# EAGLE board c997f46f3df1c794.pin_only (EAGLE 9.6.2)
REV: C

Size 80.01 x 53.34 mm. Coordinates in mm from the lower left corner, seen from the top.
Outline: 2.41,53.34 77.34,53.34 arc-90 80.01,50.93 80.01,36.32 78.23,34.92 78.23,17.27 80.01,16.13 80.01,2.54 arc-90 77.47,0 2.53,0 arc-90 0,2.53 0,50.93 arc-90 2.41,53.34
Copper layers (1*16): Top 0.035mm / dielectric 1.5mm / Bottom 0.035mm
Design rules "adafruit *": minimum track width 8mil, minimum drill 15.5mil, track to track 8mil, track to pad 8mil, pad to pad 8mil, via to via 8mil, smd to smd 8mil, copper to edge 10mil, drill to drill 8mil, minimum pad ring 10mil, minimum via ring 8mil, stop-mask expansion 2mil, vias tented up to drill 20mil, thermal gap 10mil
Net classes: 0 default: width 0.178 mm; 1 power: width 0.254 mm; 2 lowpower: width 0.305 mm, drill 0.483 mm

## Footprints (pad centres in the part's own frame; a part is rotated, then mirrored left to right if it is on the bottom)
0805-NO = smd 1.24 x 1.5: 1 -0.95,0; 2 0.95,0
0603-NO = smd 1.075 x 1: 1 -0.85,0; 2 0.85,0
CHIPLED_0603_NOOUTLINE = smd 0.8 x 0.8: A 0,-0.75; C 0,0.75
JST_SH4 = smd 0.6 x 1.55: 1 -1.5,2.514; 2 -0.5,2.514; 3 0.5,2.514; 4 1.5,2.514 | smd 1.2 x 1.8: MT1 -2.8,-1.386; MT2 2.8,-1.386
SOD-323 = smd 1.35 x 0.8: A 1.27,0; C -1.27,0
SOD-123 = smd 1.4 x 1.4: A 1.85,0; C -1.85,0
EINK_290IN = smd 1.25 x 0.275 bottom: 1 2.51,5.208; 2 2.51,4.708; 3 2.51,4.208; 4 2.51,3.708; 5 2.51,3.208; 6 2.51,2.708; 7 2.51,2.208; 8 2.51,1.708; 9 2.51,1.208; 10 2.51,0.708; 11 2.51,0.208; 12 2.51,-0.292; 13 2.51,-0.792; 14 2.51,-1.292; 15 2.51,-1.792; 16 2.51,-2.292; 17 2.51,-2.792; 18 2.51,-3.292; 19 2.51,-3.792; 20 2.51,-4.292; 21 2.51,-4.792; 22 2.51,-5.292; 23 2.51,-5.792; 24 2.51,-6.292 | smd 3 x 2 bottom: SPRT1 0.05,7.058; SPRT2 0.05,-8.052
FIDUCIAL_1MM = smd 1 x 1: 1 0,0
SOT23-6 = smd 0.55 x 1.2: 1 -0.95,-1.3; 2 0,-1.3; 3 0.95,-1.3; 4 0.95,1.3; 5 0,1.3; 6 -0.95,1.3
LGA16_3X3MM = smd 0.5 x 0.25: 1 -1.35,1; 2 -1.35,0.5; 3 -1.35,0; 4 -1.35,-0.5; 5 -1.35,-1; 9 1.35,-1; 10 1.35,-0.5; 11 1.35,0; 12 1.35,0.5; 13 1.35,1 | smd 0.25 x 0.5: 6 -0.5,-1.35; 7 0,-1.35; 8 0.5,-1.35; 14 0.5,1.35; 15 0,1.35; 16 -0.5,1.35
1X02_ROUND = drill 1 pad 1.778: 1 -1.27,0; 2 1.27,0
INDUCTOR_4X4MM_NR401 = smd 1.2 x 3.7: P$1 -1.4,0; P$2 1.4,0
WS2812B_4020 = smd 0.5 x 1.25: 1 1.3,-0.75; 2 0.45,-0.75; 3 -0.45,-0.75; 4 -1.3,-0.75
SOT23-R = smd 0.635 x 1.016: 1 -0.95,-1; 2 0.95,-1; 3 0,1
SOT23-3 = smd 0.8 x 0.9: 1 -0.95,-1; 2 0.95,-1; 3 0,1.1
0805_10MGAP = smd 1.2 x 1.5: 1 -1.05,0; 2 1.05,0
JSTPH3 = smd 1 x 4.6: 1 -2,-2.7; 2 0,-2.7; 3 2,-2.7 | smd 1.6 x 3.4: NC1 -4.4,2.5; NC2 4.4,2.5
SOLDERJUMPER_2WAY_OPEN_NOPASTE = smd 1.168 x 1.6: 1 -1.397,0; 2 0,0; 3 1.397,0
BUZZER_SMT_7.5MM = smd 2 x 2: + 2.8,-2.8; - 2.8,2.8; MT2 -2.8,2.8 | smd 2 x 1 rotated 135: MT -3,-3
SPST_TACTILE_RA = smd 1.1 x 1.5: 1 -2.1,0.9; 2 2.1,0.9 | smd 1.75 x 1: MT1 -3.175,-0.9; MT2 3.075,-0.9 | hole 1: -1.15,-0.3; 1.15,-0.3
TACTILE_3X6MM = smd 2 x 1.5: P$1 -4,0; P$2 4,0
SPDT_SMT_SSSS811101 = smd 0.7 x 1.5: A -2.25,1.75; B 0.75,1.75; C 2.25,1.75 | smd 1 x 0.8: SUP1 -3.65,1.1; SUP2 -3.65,-1.1; SUP3 3.65,1.1; SUP4 3.65,-1.1 | hole 0.9: -1.5,0; 1.5,0
TESTPOINT_ROUND_1.5MM_NO = smd 1.5 x 1.5: P$1 0,0
SMT_NUT_3MM = drill 4.25 pad 4.572: P$1 0,0
ALS-PT19-315C = smd 0.8 x 0.8: C -0.75,0; E 0.75,0
SOT23-5 = smd 0.55 x 1.2: 1 -0.95,-1.3; 2 0,-1.3; 3 0.95,-1.3; 4 0.95,1.3; 5 -0.95,1.3
MODULE_ESP32-S2-WROVER = smd 1.5 x 0.9: 1 -8.75,8; 2 -8.75,6.5; 3 -8.75,5; 4 -8.75,3.5; 5 -8.75,2; 6 -8.75,0.5; 7 -8.75,-1; 8 -8.75,-2.5; 9 -8.75,-4; 10 -8.75,-5.5; 11 -8.75,-7; 12 -8.75,-8.5; 13 -8.75,-10; 14 -8.75,-11.5; 15 -8.75,-13; 16 -8.75,-14.5; 27 8.75,-14.5; 28 8.75,-13; 29 8.75,-11.5; 30 8.75,-10; 31 8.75,-8.5; 32 8.75,-7; 33 8.75,-5.5; 34 8.75,-4; 35 8.75,-2.5; 36 8.75,-1; 37 8.75,0.5; 38 8.75,2; 39 8.75,3.5; 40 8.75,5; 41 8.75,6.5; 42 8.75,8 | smd 0.9 x 1.5: 17 -6.75,-15.25; 18 -5.25,-15.25; 19 -3.75,-15.25; 20 -2.25,-15.25; 21 -0.75,-15.25; 22 0.75,-15.25; 23 2.25,-15.25; 24 3.75,-15.25; 25 5.25,-15.25; 26 6.75,-15.25 | smd 1.1 x 1.1: 43_1 -2.69,1.45; 43_2 -1.19,1.45; 43_3 0.31,1.45; 43_4 -2.69,-0.05; 43_5 -1.19,-0.05; 43_6 0.31,-0.05; 43_7 -2.69,-1.55; 43_8 -1.19,-1.55; 43_9 0.31,-1.55 | drill 0.4: 43_10 -1.94,1.45; 43_11 -0.44,1.45; 43_12 -2.69,0.7; 43_13 -1.19,0.7; 43_14 0.31,0.7; 43_15 -1.94,-0.05; 43_16 -0.44,-0.05; 43_17 -2.69,-0.8; 43_18 -1.19,-0.8; 43_19 0.31,-0.8; 43_20 -1.94,-1.55; 43_21 -0.44,-1.55
JSTPH2_BATT = smd 1 x 4.6: 1 -1,-3.7; 2 1,-3.7 | smd 1.6 x 3.4: NC1 -3.4,1.5; NC2 3.4,1.5
USB_C_CUSB31-CFM2AX-01-X = smd 0.575 x 1.15: A1B12 -3.2,3.545; A4B9 -2.4,3.545; B1A12 3.2,3.545; B4A9 2.4,3.545 | smd 0.275 x 1.15: A5 -1.25,3.545; A6 -0.25,3.545; A7 0.25,3.545; A8 1.25,3.545; B5 1.75,3.545; B6 0.75,3.545; B7 -0.75,3.545; B8 -1.75,3.545 | drill 0.6 pad 1 long: M1 -4.32,2.97; M2 4.32,2.97; M3 -4.32,-1.21; M4 4.32,-1.21 | hole 0.65: 2.89,2.47; -2.89,2.47

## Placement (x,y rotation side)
C1  10uF  [0805-NO]  8.45,15.68 90 top
C2  0.1uF  [0603-NO]  65.6,34.67 0 top
C3  10µF  [0805-NO]  30.1,46.61 270 top
C4  10µF  [0805-NO]  22.35,15.11 0 top
C5  0.1uF  [0603-NO]  22.48,13.34 0 top
C6  1uF  [0603-NO]  28.19,33.08 90 top
C7  10µF  [0805-NO]  5.08,43.31 180 top
C8  10µF  [0805-NO]  69.6,6.41 180 top
C9  10uF/10V+  [0805-NO]  65.62,36.32 180 top
C10  10µF  [0805-NO]  5.08,45.21 180 top
C11  10µF  [0805-NO]  19.11,9.78 180 top
C12  1uF  [0603-NO]  68.9,47.75 0 top
C13  10µF  [0805-NO]  18.03,15.94 180 top
C14  1uF  [0603-NO]  2.79,20.26 270 top
C15  0.1uF  [0603-NO]  10.29,15.75 90 top
C16  0.1uF  [0603-NO]  65.98,4.76 0 top
C17  10µF  [0805-NO]  5.21,41.4 180 top
C18  10µF  [0805-NO]  63.25,27.75 180 top
C19  1uF  [0805-NO]  72.35,40.6 0 top
C20  10uF  [0805-NO]  49.78,4 270 top
C21  0.1uF  [0603-NO]  15.05,19.94 270 top
C23  1uF  [0805-NO]  63.25,25.78 0 top
C24  1uF  [0805-NO]  63.25,21.97 0 top
C25  1uF  [0805-NO]  63.25,20.07 0 top
C26  1uF  [0805-NO]  63.25,18.16 0 top
C27  1uF  [0805-NO]  69.47,36.58 180 top
C28  1uF  [0805-NO]  62.87,42.86 0 top
C29  4.7uF/25V  [0805-NO]  66.8,42.8 180 top
C30  1uF  [0805-NO]  72.26,38.61 0 top
C31  1uF  [0805-NO]  63.25,23.88 0 top
CHG1  ORANGE  [CHIPLED_0603_NOOUTLINE]  11.87,2.35 0 top
CONN1  STEMMA_I2C_QT  [JST_SH4]  40.64,2.79 0 top
D1  3.6V  [SOD-323]  30.86,6.86 0 top
D2  MBR0530  [SOD-123]  63.82,46.86 0 top
D3  MBR0530  [SOD-123]  63.88,44.96 180 top
D4  MBR540  [SOD-123]  13.65,14.61 180 top
D5  MBR0530  [SOD-123]  69.6,40.89 90 top
D6  3.6V  [SOD-323]  49.28,8 0 top
EINK2  EINK_24PIN_290IN  [EINK_290IN]  69.88,26.57 0 bottom
FID1  FIDUCIAL_1MM  [FIDUCIAL_1MM]  0.97,45.97 0 top
FID2  FIDUCIAL_1MM  [FIDUCIAL_1MM]  7.48,1.09 90 top
FID3  FIDUCIAL_1MM  [FIDUCIAL_1MM]  77.98,43.81 0 top
FID4  FIDUCIAL_1MM  [FIDUCIAL_1MM]  74.8,9.65 0 bottom
FID5  FIDUCIAL_1MM  [FIDUCIAL_1MM]  77.98,43.81 0 bottom
FID6  FIDUCIAL_1MM  [FIDUCIAL_1MM]  8.64,6.35 0 bottom
IC2  PAM8301  [SOT23-6]  33.91,10.41 270 top
IC4  LIS3DH  [LGA16_3X3MM]  40.77,10.48 180 top
JP2  UART  [1X02_ROUND]  28.07,39.12 90 top
L  RED  [CHIPLED_0603_NOOUTLINE]  14.29,2.29 180 top
L1  10uH  [INDUCTOR_4X4MM_NR401]  66.04,39.5 180 top
LED2  WS2812B_4020  [WS2812B_4020]  15.88,49.53 180 bottom
LED3  WS2812B_4020  [WS2812B_4020]  31.75,49.53 180 bottom
LED4  WS2812B_4020  [WS2812B_4020]  48.26,49.53 180 bottom
LED5  WS2812B_4020  [WS2812B_4020]  64.77,49.53 180 bottom
ON  GREEN  [CHIPLED_0603_NOOUTLINE]  16.57,2.29 180 top
Q1  DMG3415U-7  [SOT23-R]  12.32,11.68 270 top
Q2  DMG3415  [SOT23-R]  21.97,17.78 270 top
Q3  DMG3415U-7  [SOT23-R]  15.94,11.94 270 top
Q5  IRLML0100  [SOT23-3]  68.45,45.34 90 top
R1  10K  [0603-NO]  5.27,21.46 0 top
R2  10K  [0603-NO]  11.81,5.46 90 top
R3  5.1K  [0603-NO]  9.53,9.72 180 top
R4  5.1k  [0603-NO]  65.98,2.98 180 top
R5  10K  [0603-NO]  44.58,4.06 90 top
R6  47K  [0603-NO]  16.32,5.4 90 top
R7  10K  [0603-NO]  36.7,4.19 90 top
R8  5.1K  [0603-NO]  9.21,13.4 180 top
R9  10K  [0603-NO]  14.16,5.46 90 top
R10  1Meg  [0603-NO]  63.63,5.46 270 top
R11  1Meg  [0603-NO]  65.98,6.35 0 top
R12  100k  [0603-NO]  14.67,9.65 0 top
R13  0.47ohm  [0805_10MGAP]  72.71,42.67 180 top
R14  100k  [0603-NO]  9.46,8.13 180 top
R15  100K  [0603-NO]  22.1,20.19 0 top
R16  1K  [0603-NO]  29.21,9.02 0 top
R17  1Meg  [0603-NO]  28.13,29.91 90 top
R18  1K  [0603-NO]  49.28,9.53 180 top
R19  47K  [0603-NO]  17.34,17.97 0 top
R20  10K  [0603-NO]  5.59,36.39 90 top
R21  DNP  [0805_10MGAP]  71.88,45.47 270 top
R22  DNP  [0603-NO]  29.59,3.3 270 top
R23  DNP  [0603-NO]  46.1,4.06 270 top
R24  DNP  [0603-NO]  6.03,25.21 270 top
R25  DNP  [0603-NO]  62.1,5.46 90 top
R26  100K  [0603-NO]  34.48,8 0 top
R27  100K  [0603-NO]  63.18,29.53 0 top
SENSE  JST PH 3  [JSTPH3]  23.62,4.57 180 top
SENSE1  JST PH 3  [JSTPH3]  56.39,4.57 180 top
SJ2  [SOLDERJUMPER_2WAY_OPEN_NOPASTE]  33.15,1.52 0 top
SP1  7.5mm SPK  [BUZZER_SMT_7.5MM]  27.94,15.88 270 top
SW1  RA_TACT  [SPST_TACTILE_RA]  1.78,38.1 270 top
SW2  [TACTILE_3X6MM]  15.24,3.81 0 bottom
SW3  RA_TACT  [SPST_TACTILE_RA]  1.78,25.4 270 top
SW4  SPDT R/A  [SPDT_SMT_SSSS811101]  67.31,51.56 180 top
SW5  [TACTILE_3X6MM]  31.75,3.81 0 bottom
SW6  [TACTILE_3X6MM]  48.26,3.81 0 bottom
SW7  [TACTILE_3X6MM]  64.77,3.81 0 bottom
TP1  [TESTPOINT_ROUND_1.5MM_NO]  1.27,43.18 270 top
TP2  SEWTAP_SMTNUTM3  [SMT_NUT_3MM]  3.81,49.53 0 top
TP3  SEWTAP_SMTNUTM3  [SMT_NUT_3MM]  3.81,3.81 0 top
TP4  SEWTAP_SMTNUTM3  [SMT_NUT_3MM]  76.2,49.53 0 top
TP5  SEWTAP_SMTNUTM3  [SMT_NUT_3MM]  76.2,3.81 0 top
TP6  [TESTPOINT_ROUND_1.5MM_NO]  1.27,20.32 0 top
TP7  [TESTPOINT_ROUND_1.5MM_NO]  1.27,20.32 0 bottom
TP8  [TESTPOINT_ROUND_1.5MM_NO]  1.27,43.18 0 bottom
U1  [ALS-PT19-315C]  40.01,50.8 0 bottom
U2  MCP73831T-2ACI/OT  [SOT23-5]  69.6,3.75 90 top
U3  ESP32-S2-WROVER  [MODULE_ESP32-S2-WROVER]  17.46,37.85 0 top
U4  AP2112K-3.3  [SOT23-5]  19.18,12.83 0 top
U$15  [PCBFEAT-REV-040]  1.59,32 0 top
U$69  [MAGTAG_BOTTOM]  80.01,0 0 bottom
U$70  [MAGTAG_FRONT]  0,0 0 top
X1  JSTPH  [JSTPH2_BATT]  70.42,11.68 90 top
X4  USB C  [USB_C_CUSB31-CFM2AX-01-X]  2.92,12.7 270 top

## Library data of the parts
C1-C21 C23-C31 CHG1 CONN1 D1-D6 EINK2 IC2 IC4 JP2 L L1 LED2-LED5 ON Q1-Q3 R1-R27 SENSE SENSE1 SJ2 SP1 SW1-SW7 TP1-TP8 U1 U2 U4 U$15 X1 X4 = microbuilder
FID1-FID6 = microbuilder; BOM: EXCLUDE
Q5 = Parts
U3 = adafruit_wireless; AVAILABILITY: Warning; DESCRIPTION: WiFi 802.11b/g/n Transceiver Module 2.4GHz Antenna Not Included Surface Mount; DIGIKEY-PURCHASE-URL: https://snapeda.com/shop?store=DigiKey&id=4614060; MF: Espressif Systems; MP: ESP32-S2-WROVER; PACKAGE: VFQFN-56 Espressif Systems; PRICE: None
U$69 U$70 = portal_silks

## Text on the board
214bmp: D:/SmartProjects/Snc/a4_bn_logo2.bmp

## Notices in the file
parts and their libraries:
microbuilder: This work is placed in the public domain, and may be freely used for commercial and non-commercial work with the following conditions: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
